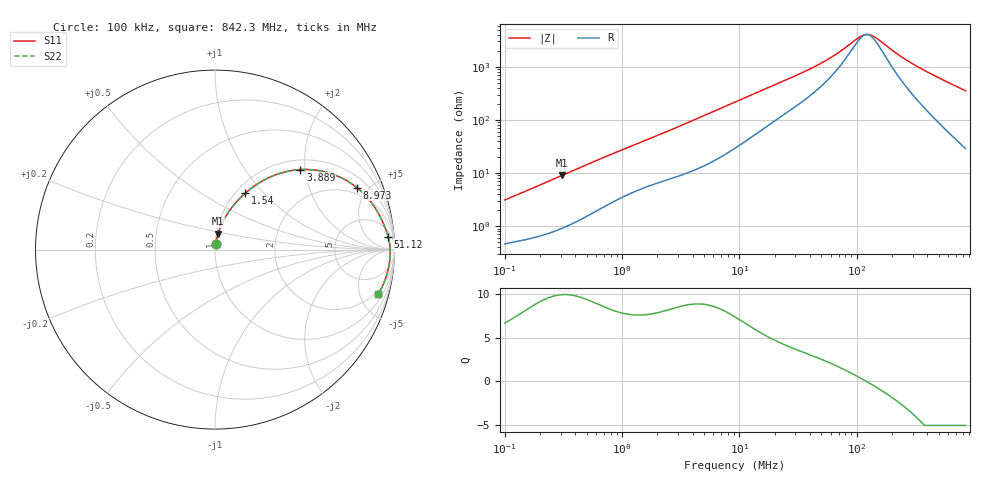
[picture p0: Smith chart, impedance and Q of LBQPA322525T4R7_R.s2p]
! LBQPA322525T4R7_R  S-PARAMETER MODEL  ( General Type )
! Model Generated by TAIYO YUDEN Corporation (http://www.ty-top.com)
! Version 1.0
! TAIYO YUDEN Control No. 191025NI43SB-FBB
! Copyright(c) 2019 TAIYO YUDEN CO.,LTD. All Rights Reserved.
! Product Description (link to TY-COMPAS)
! https://ds.yuden.co.jp/TYCOMPAS/or/detail?pn=LBQPA322525T4R7MR&u=M
! Products Name : Inductors
! Characteristics :
!  Inductance : 4.7 uH , SRF(min) : 70 MHz , DC Resistance(max) : 0.13 Ohm
!  Rated Current : Saturation :1250 mA , Temp Rise : 830 mA (20 degC)
!  Case Size : 3.2 x 2.5 / 0.126 x 0.098 [mm/inch] , Thickness : 2.5 / 0.098 [mm/inch]
!  (Conditions: Temperature = 25 degC , DC Bias Current/Voltage = 0A / 0V)
! External Node Assignments :
!  1  o---GGG---o  2
! GND o---------o GND
! Frequency Range : 0.1MHz  -  842.342835MHz  [ 402 STEP ]
# MHz S RI R 50
! Freq[MHz].  S11 Real  S11 Imag  S21 Real  S21 Imag  S12 Real  S12 Imag  S22 Real  S22 Imag
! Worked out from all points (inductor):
!   401 points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, 100 kHz to 842.3 MHz, reference 50 ohm
!   read as one part in series: L = 4.81 uH near 104.6 kHz
!   highest Q = 9.88 at 309.5 kHz (marker M1), where L = 4.65 uH
!   self-resonance near 121.2 MHz
!   S11 on the Smith chart (normalised r, x): 100 kHz: 1.01, +0.06; 1.54 MHz: 1.11, +0.80; 3.889 MHz: 1.21, +1.88; 8.973 MHz: 1.57, +4.22; 51.12 MHz: 10, +22; 842.3 MHz: 1.58, -7.10
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0.1  0.00555 0.0305  0.9945 -0.0305  0.9945 -0.0305  0.00555 0.0305
0.309518  0.0169 0.088  0.9831 -0.088  0.9831 -0.088  0.0169 0.088
0.454485  0.0296 0.1251  0.9704 -0.1251  0.9704 -0.1251  0.0296 0.1251
0.87522  0.0792 0.2148  0.9208 -0.2148  0.9208 -0.2148  0.0792 0.2148
1.539786  0.1693 0.3148  0.8307 -0.3148  0.8307 -0.3148  0.1693 0.3148
2.065565  0.2427 0.3698  0.7573 -0.3698  0.7573 -0.3698  0.2427 0.3698
3.888866  0.4763 0.4457  0.5237 -0.4457  0.5237 -0.4457  0.4763 0.4457
5.710265  0.6383 0.426  0.3617 -0.426  0.3617 -0.426  0.6383 0.426
8.972856  0.7894 0.346  0.2106 -0.346  0.2106 -0.346  0.7894 0.346
9.177924  0.7953 0.3412  0.2047 -0.3412  0.2047 -0.3412  0.7953 0.3412
16.89332  0.9019 0.2165  0.0981 -0.2165  0.0981 -0.2165  0.9019 0.2165
41.71227  0.9587 0.0917  0.0413 -0.0917  0.0413 -0.0917  0.9587 0.0917
51.11959  0.9647 0.0715  0.0353 -0.0715  0.0353 -0.0715  0.9647 0.0715
70.14221  0.9711 0.0434  0.0289 -0.0434  0.0289 -0.0434  0.9711 0.0434
102.9942  0.9752 0.0126  0.0248 -0.0126  0.0248 -0.0126  0.9752 0.0126
117.9492  0.9759 0.00213  0.0241 -0.00213  0.0241 -0.00213  0.9759 0.00213
129.107  0.9762 -0.00489  0.0238 0.00489  0.0238 0.00489  0.9762 -0.00489
141.3204  0.9763 -0.012  0.0237 0.012  0.0237 0.012  0.9763 -0.012
189.5759  0.9757 -0.0361  0.0243 0.0361  0.0243 0.0361  0.9757 -0.0361
248.6268  0.9735 -0.061  0.0265 0.061  0.0265 0.061  0.9735 -0.061
348.9424  0.9675 -0.0983  0.0325 0.0983  0.0325 0.0983  0.9675 -0.0983
842.3428  0.9096 -0.2488  0.0904 0.2488  0.0904 0.2488  0.9096 -0.2488
